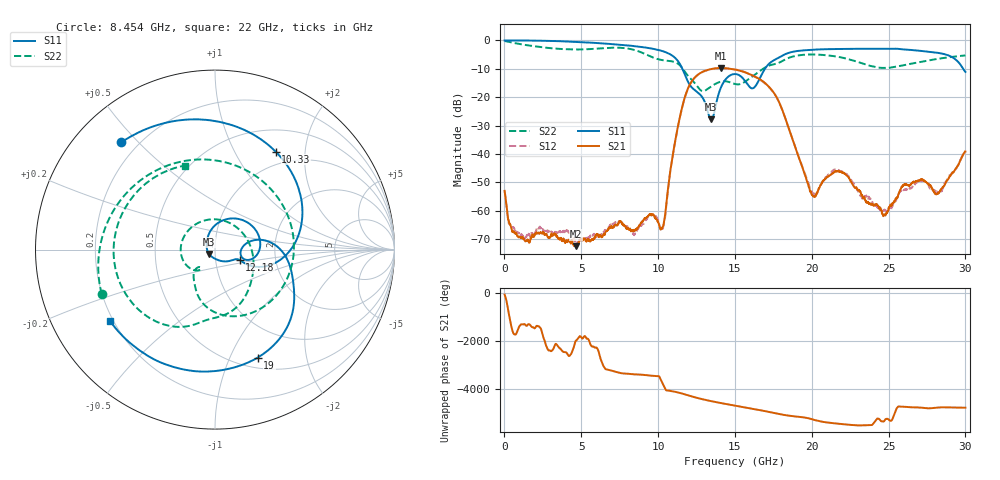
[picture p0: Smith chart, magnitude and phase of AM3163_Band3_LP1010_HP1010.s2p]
!Agilent Technologies,E8364B,MY43040894,A.07.50.67
!Agilent E8364B: A.07.50.67
!Date: Thursday, August 20, 2020 11:08:47
!Correction: S11(Full 2 Port(1,2))
!S21(Full 2 Port(1,2))
!S12(Full 2 Port(1,2))
!S22(Full 2 Port(1,2))
!S2P File: Measurements: S11, S21, S12, S22:
# Hz S  dB  R 50
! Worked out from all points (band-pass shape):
!   3201 points, 10 MHz to 30 GHz, reference 50 ohm
!   highest |S21| = -9.73 dB at 14.1 GHz (marker M1); lowest = -72.4 dB at 4.63 GHz (marker M2)
!   |S21| within 3 dB of the highest: 12.45 GHz to 16.3 GHz (3.849 GHz wide, 26.8 % of centre)
!   lowest |S11| = -27.8 dB at 13.45 GHz (marker M3), VSWR 1.09, Z = 46.8 - j2.3 ohm
!   |S11| at or under -10 dB: 11.58 GHz to 16.95 GHz (5.372 GHz wide, 37.7 % of centre); 29.85 GHz to end of sweep
!   |S22| runs from -17.9 to -0.2 dB; largest |S21 - S12| = 0.0068
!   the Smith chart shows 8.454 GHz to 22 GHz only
!   S11 on the Smith chart (normalised r, x): 8.454 GHz: 0.14, +0.45; 10.33 GHz: 0.80, +1.48; 12.18 GHz: 1.31, -0.16; 19 GHz: 0.62, -1.28; 22 GHz: 0.19, -0.30
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1e7  -0.03 -1.8  -52.95 -53.4  -52.83 22.6  -0.23 -5.9
1.087766e9  -0.05 -29.5  -69.21 135.4  -68.44 -143.4  -1.36 -82.3
2.381084e9  -0.13 -64.3  -67.78 -57.5  -66.14 -70.9  -2.37 -161.5
4.630334e9  -0.53 -123.3  -72.42 154.4  -70.29 129.6  -3.20 80.0
5.014581e9  -0.62 -133.2  -70.18 -62.5  -69.76 -75.9  -3.18 59.4
6.195438e9  -1.00 -164.1  -68.83 -80.2  -68.55 -89.9  -2.84 -7.2
7.254459e9  -1.40 167.1  -64.85 -52.2  -64.13 -53.1  -2.56 -72.8
8.454059e9  -2.01 131.1  -66.91 -161.2  -68.23 -157.6  -3.37 -158.5
1.000979e10  -3.36 73.1  -64.01 125.0  -63.34 108.1  -6.64 57.4
1.032843e10  -3.85 58.2  -65.27 133.6  -65.80 -31.9  -6.99 24.0
1.129374e10  -7.29 1.9  -30.16 162.8  -30.39 162.8  -8.22 -73.1
1.218407e10  -16.51 -22.9  -14.45 -3.6  -14.56 -3.0  -13.83 -125.5
1.344927e10  -27.78 -143.1  -10.09 158.8  -10.14 159.1  -16.20 -131.1
1.409593e10  -16.49 83.3  -9.73 76.3  -9.84 76.9  -14.50 -162.7
1.5005e10  -11.83 13.5  -10.25 -30.8  -10.21 -29.7  -15.35 102.3
1.744169e10  -7.29 -13.4  -17.77 37.7  -17.88 39.1  -8.52 -86.7
1.899742e10  -3.78 -68.4  -38.71 -127.6  -38.68 -125.5  -5.41 -138.8
2.000958e10  -3.28 -98.0  -54.29 121.1  -53.25 114.7  -4.95 -175.6
2.199642e10  -3.01 -145.5  -46.61 -88.6  -46.22 -87.7  -6.08 109.4
2.500479e10  -3.01 145.2  -58.89 112.2  -59.42 -48.5  -9.66 -53.1
2.735713e10  -3.85 79.6  -49.65 -130.9  -49.63 -131.8  -7.30 -162.1
3e10  -11.10 -23.5  -39.12 -118.8  -38.83 -118.4  -5.30 111.4
